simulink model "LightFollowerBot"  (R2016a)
settings: Solver=FixedStepAuto  StartTime=0.0  StopTime=inf  RelTol=1e-3
libraries: miniQ x3

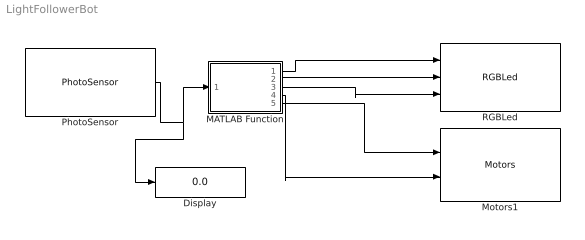
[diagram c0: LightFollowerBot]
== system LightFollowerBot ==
  Display : Display
  MATLAB Function : MATLAB Function  TreatAsAtomicUnit=on
  Motors1 : miniQ/Motors  flipLeft=off  flipRight=off
  PhotoSensor : miniQ/PhotoSensor  sampleTime_dd=0.01  debug_dd=off
  RGBLed : miniQ/RGBLed
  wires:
  MATLAB Function/3(blue) -> RGBLed/3
  MATLAB Function/1(red) -> RGBLed/1
  MATLAB Function/2(green) -> RGBLed/2
  PhotoSensor/1 -> Display/1, MATLAB Function/1(lite)
  MATLAB Function/4(MR) -> Motors1/2
  MATLAB Function/5(ML) -> Motors1/1

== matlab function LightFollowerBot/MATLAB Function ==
function [red,green,blue,MR,ML] = fcn(lite)

if lite<100
        MR=100;
        ML=-100;
        
        red=0;
        green=255;
        blue=0;
elseif lite>900
        MR=-100;
        ML=100;
        
        red=0;
        green=0;
        blue=255;
else
        MR=100;
        ML=100;
        
        red=255;
        green=0;
        blue=255;
end
end
